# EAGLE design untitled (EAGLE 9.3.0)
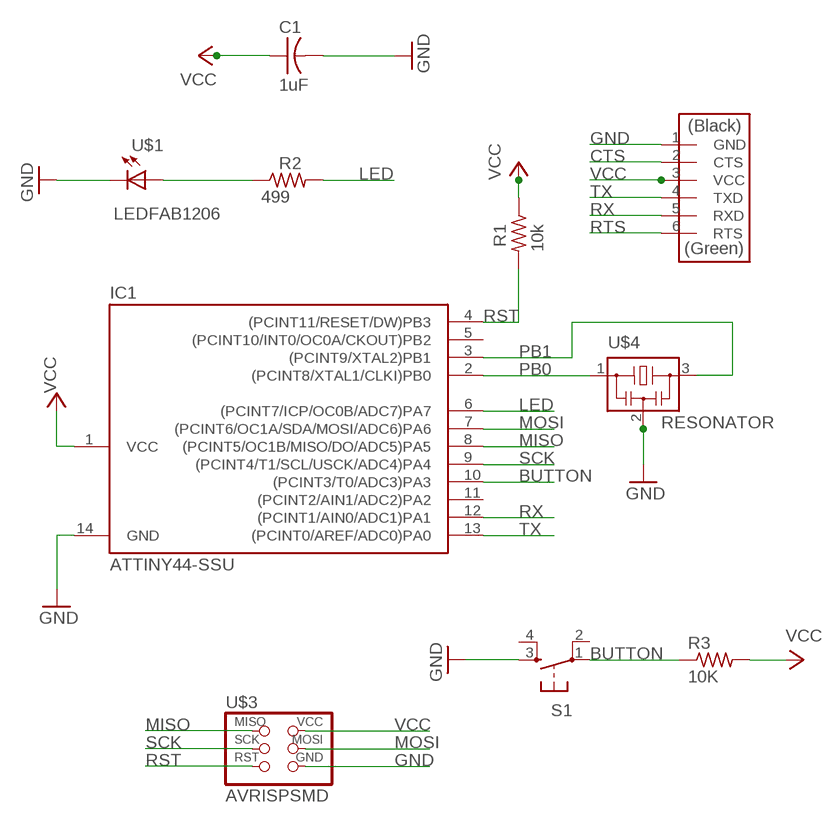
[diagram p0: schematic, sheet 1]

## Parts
C1  1uF  CAP-US1206FAB  [C1206FAB]
IC1  ATTINY44-SSU  [SOIC14]
R1  10k  RES-US1206FAB  [R1206FAB]
R2  499  RES-US1206FAB  [R1206FAB]
R3  10K  RES-US1206FAB  [R1206FAB]
S1  6MM_SWITCH6MM_SWITCH  [6MM_SWITCH]
U$1  LEDFAB1206  [LED1206FAB]
U$2  FTDI-SMD-HEADER  [1X06SMD]
U$3  AVRISPSMD  [2X03SMD]
U$4  RESONATOR  [EFOBM]

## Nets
BUTTON: IC1.10((PCINT3/T0/ADC3)PA3) R3.1 S1.1(P)
CTS: U$2.2(CTS)
GND: C1.2 IC1.14(GND) S1.3(S) U$1.2(C) U$2.1(GND) U$3.6(GND) U$4.2
LED: IC1.6((PCINT7/ICP/OC0B/ADC7)PA7) R2.2
MISO: IC1.8((PCINT5/OC1B/MISO/DO/ADC5)PA5) U$3.1(MISO)
MOSI: IC1.7((PCINT6/OC1A/SDA/MOSI/ADC6)PA6) U$3.4(MOSI)
N$4: R2.1 U$1.1(A)
PB0: IC1.2((PCINT8/XTAL1/CLKI)PB0) U$4.1
PB1: IC1.3((PCINT9/XTAL2)PB1) U$4.3
RST: IC1.4((PCINT11/RESET/DW)PB3) R1.2 U$3.5(RST)
RTS: U$2.6(RTS)
RX: IC1.12((PCINT1/AIN0/ADC1)PA1) U$2.5(RXD)
SCK: IC1.9((PCINT4/T1/SCL/USCK/ADC4)PA4) U$3.3(SCK)
TX: IC1.13((PCINT0/AREF/ADC0)PA0) U$2.4(TXD)
VCC: C1.1 IC1.1(VCC) R1.1 R3.2 U$2.3(VCC) U$3.2(VCC)
Unconnected: IC1.5((PCINT10/INT0/OC0A/CKOUT)PB2) IC1.11((PCINT2/AIN1/ADC2)PA2) S1.2(P1) S1.4(S1)

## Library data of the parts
C1 = fab:CAP-US
IC1 = fab:ATTINY44
R1-R3 = fab:RES-US: Resistor (US Symbol)
S1 = fab:6MM_SWITCH: OMRON SWITCH
U$1 = fab:LED: LED
U$2 = fab:FTDI-SMD-HEADER
U$3 = fab:AVRISP
U$4 = fab:RESONATOR

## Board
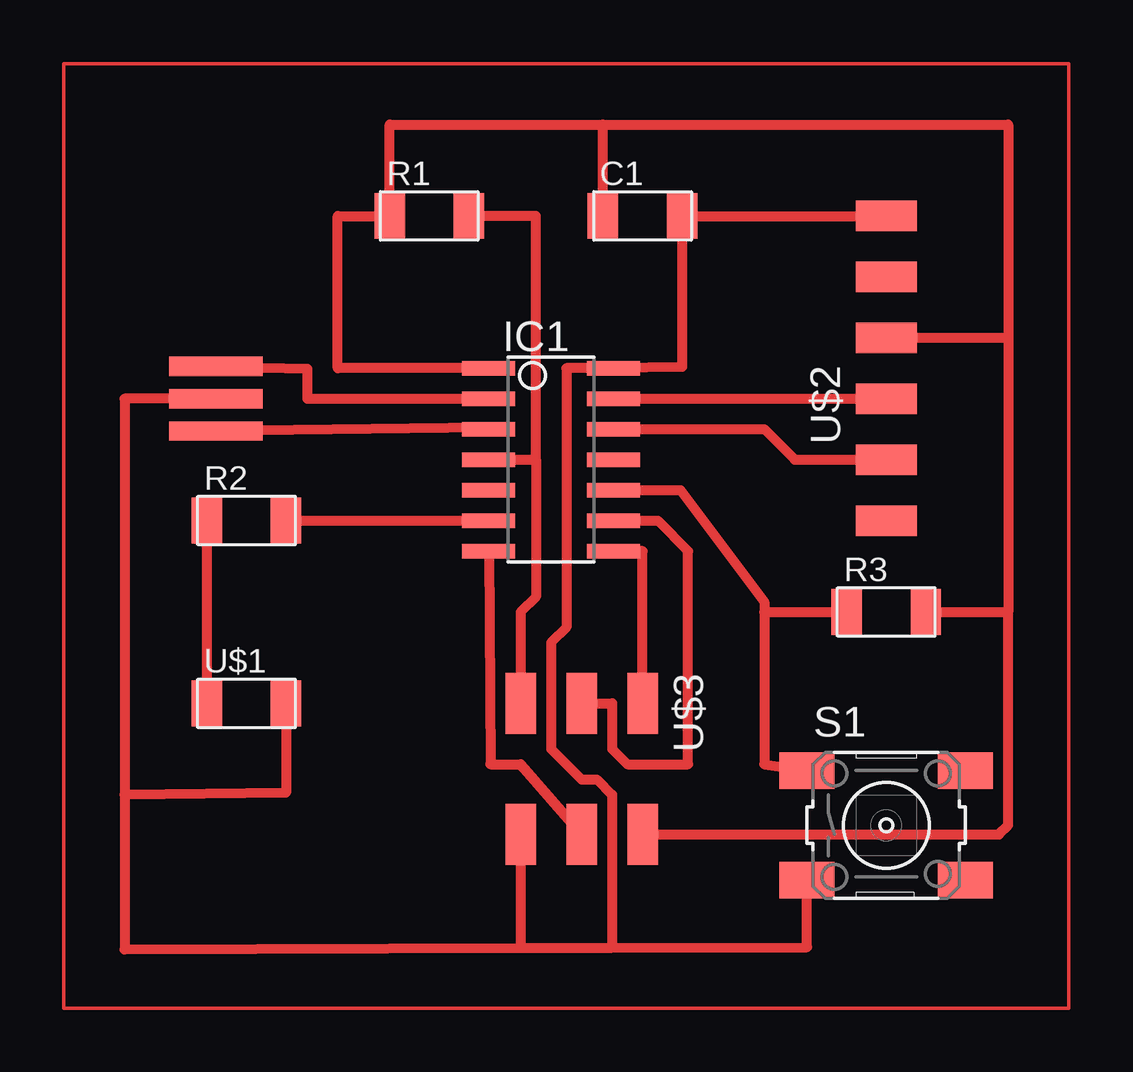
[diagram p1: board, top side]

No outline drawn. Coordinates in mm, seen from the top.
Copper layers (1*16): Top 0.035mm / dielectric 1.5mm / Bottom 0.035mm
Design rules "default *": minimum track width 16mil, minimum drill 0.35mm, track to track 6mil, track to pad 6mil, pad to pad 6mil, via to via 6mil, smd to smd 6mil, copper to edge 40mil, drill to drill 6mil, minimum pad ring 10mil, minimum via ring 8mil, stop-mask expansion 4mil, vias tented up to drill 0mil, thermal gap 10mil

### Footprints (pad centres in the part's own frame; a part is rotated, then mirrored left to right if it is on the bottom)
C1206FAB = smd 1.27 x 1.905: 1 -1.651,0; 2 1.651,0
SOIC14 = smd 0.61 x 2.21: 1 -3.81,-2.603; 2 -2.54,-2.603; 3 -1.27,-2.603; 4 0,-2.603; 5 1.27,-2.603; 6 2.54,-2.603; 7 3.81,-2.603; 8 3.81,2.603; 9 2.54,2.603; 10 1.27,2.603; 11 0,2.603; 12 -1.27,2.603; 13 -2.54,2.603; 14 -3.81,2.603
R1206FAB = smd 1.27 x 1.905: 1 -1.651,0; 2 1.651,0
6MM_SWITCH = smd 2.286 x 1.524: 1 -3.302,2.286; 2 3.302,2.286; 3 -3.302,-2.286; 4 3.302,-2.286
LED1206FAB = smd 1.27 x 1.905: 1 -1.651,0; 2 1.651,0
1X06SMD = smd 2.54 x 1.27: 1 0,6.35; 2 0,3.81; 3 0,1.27; 4 0,-1.27; 5 0,-3.81; 6 0,-6.35
2X03SMD = smd 2.54 x 1.27: 1 -2.54,2.54; 2 2.92,2.54; 3 -2.54,0; 4 2.92,0; 5 -2.54,-2.54; 6 2.92,-2.54
EFOBM = smd 0.8 x 3.9: 1 -1.35,0; 2 0,0; 3 1.35,0

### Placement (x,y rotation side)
C1  15.24,45.72 0 top
IC1  11.43,35.56 270 top
R1  6.35,45.72 0 top
R2  -1.27,33.02 0 top
R3  25.4,29.21 0 top
S1  25.4,20.32 0 top
U$1  -1.27,25.4 0 top
U$2  25.4,39.37 0 top
U$3  12.7,22.86 270 top
U$4  -2.54,38.1 270 top

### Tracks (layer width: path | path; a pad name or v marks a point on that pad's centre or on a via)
BUTTON
  Top 0.406: IC1.10 16.83,34.29 20.32,29.63 20.32,29.21 | 20.32,29.21 R3.1 | 20.32,29.21 20.32,22.86 S1.1
GND
  Top 0.406: U$2.1 C1.2 16.89,39.42 IC1.14 12.06,39.37 12.06,28.57 11.43,27.94 11.43,23.5 12.7,22.23 13.34,22.23 13.97,21.59 13.97,15.21 | U$4.2 -6.35,38.1 -6.35,21.59 | -6.35,21.59 -6.35,15.15 10.16,15.2 | 10.16,15.2 13.97,15.21 | 13.97,15.21 22.1,15.24 S1.3 | U$3.6 10.16,15.2 | U$1.2 0.38,21.68 -6.35,21.59
LED
  Top 0.406: R2.2 IC1.6
MISO
  Top 0.406: U$3.1 15.24,31.75 IC1.8
MOSI
  Top 0.406: IC1.7 8.9,22.86 10.16,22.86 U$3.4
N$1
  Top 0.152: -8.89,52.07 -8.89,12.7 33.02,12.7 33.02,52.07 -8.89,52.07
N$4
  Top 0.406: R2.1 U$1.1
PB0
  Top 0.406: U$4.1 -2.51,39.42 1.27,39.34 1.27,38.1 IC1.2
PB1
  Top 0.406: IC1.3 8.76,36.89 U$4.3
RST
  Top 0.406: 10.79,35.56 10.79,45.72 R1.2 | IC1.4 10.79,35.56 | 10.79,35.56 10.79,29.84 10.16,29.21 U$3.5
RX
  Top 0.406: IC1.12 20.32,36.83 21.59,35.56 U$2.5
SCK
  Top 0.406: 12.83,25.4 U$3.3 13.97,25.4 13.97,23.5 14.61,22.86 17.14,22.86 17.14,31.75 15.88,33.02 IC1.9
TX
  Top 0.406: IC1.13 U$2.4
VCC
  Top 0.406: IC1.1 2.54,39.37 2.54,45.72 R1.1 4.7,49.53 13.59,49.53 | 30.48,40.64 30.48,49.53 13.59,49.53 | 30.48,40.64 30.48,29.21 | 30.48,29.21 30.48,20.32 30.1,19.94 U$3.2 | R3.2 30.48,29.21 | C1.1 13.59,49.53 | U$2.3 30.48,40.64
